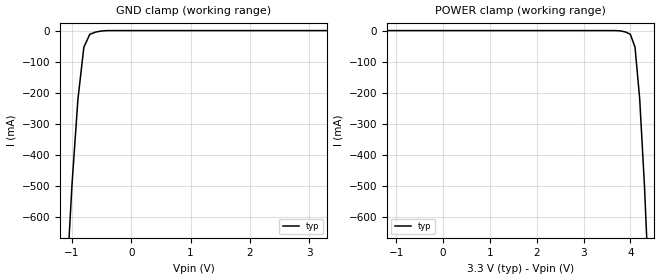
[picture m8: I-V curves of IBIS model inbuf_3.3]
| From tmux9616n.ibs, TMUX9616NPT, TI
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| inbuf_3.3
[Model]   inbuf_3.3
Model_type   Input
Vinl = 0.99
Vinh = 1.98
|   typ   min   max
C_comp   1.598234e-12   NA   NA
[Voltage Range]   3.3   NA   NA
[Temperature Range]   27   NA   NA
[Power Clamp Reference]   3.3   NA   NA
[GND Clamp Reference]   0   NA   NA
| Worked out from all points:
|   GND clamp passes 1 mA (typ) near -0.48 V on its own axis
[GND Clamp]
|   Voltage   I(typ)   I(min)   I(max)
-6.6V     -25.28A    NA         NA
-1.1V     -840.5mA   NA         NA
-1V       -493.7mA   NA         NA
-900mV    -220.1mA   NA         NA
-800mV    -53.38mA   NA         NA
-700mV    -11.97mA   NA         NA
-600mV    -4.747mA   NA         NA
-400mV    -114.3uA   NA         NA
3.3V      347.8nA    NA         NA
[POWER Clamp]
|   Voltage   I(typ)   I(min)   I(max)
-3.3V     695.6nA    NA         NA
3.6V      -5.2uA     NA         NA
3.8V      -1.179mA   NA         NA
3.9V      -4.747mA   NA         NA
4V        -11.97mA   NA         NA
4.1V      -53.38mA   NA         NA
4.2V      -220.1mA   NA         NA
4.3V      -493.7mA   NA         NA
4.4V      -840.5mA   NA         NA
6.6V      -10.26A    NA         NA
